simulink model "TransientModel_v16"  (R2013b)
settings: Solver=ode4  StartTime=0.0  StopTime=1500  FixedStep=0.001  RelTol=1e-3
InitFcn:
  | Init_model
StopFcn:
  | Postprocessing2
  | %export_results
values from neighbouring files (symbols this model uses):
  dP = (0:0.005:1)'    [CurveFit_v6_trans.m]
  dP_drag = (0:0.005:1)'    [CurveFit_v6_drag.m]
  Pboost_vec_spd = n_un    [Init_steady_maps.m]
  Pboost_vec_Thr = M_un    [Init_steady_maps.m]
  Pedal = 90    [CurveFit_v6_drag.m]    (also in CurveFit_v6_trans.m = 0:10:90)
  t_sample = 0.01    [Init_model.m]
  time_dy = 0:0.01:5    [CurveFit_v6_drag.m]    (also in CurveFit_v6_trans.m = 0:0.01:10)
undefined symbols (not defined in the file or in its folder): dtaf_sub, dtMbu_sub, dtmf_sub, dtPboost_sub, dtSpeed_Turb_sub, dY, dY_af, dY_af_drag, dY_drag, dY_Mbu, dY_Mbu_drag, dY_mf, dY_mf_drag, dY_Speed_Turb, dY_Speed_Turb_drag, EngineSpeed, EngineSpeed_vec_LM, Mbu_sub_end, Mode, Pboost_Matrix, Speed, Table, Throttle_init, time_dP, time_dP_drag, time_dy_drag, Time_LM, Time_simple, Time_SM, Time_vec_LM
libraries: simulink x45, simulink_extras x4
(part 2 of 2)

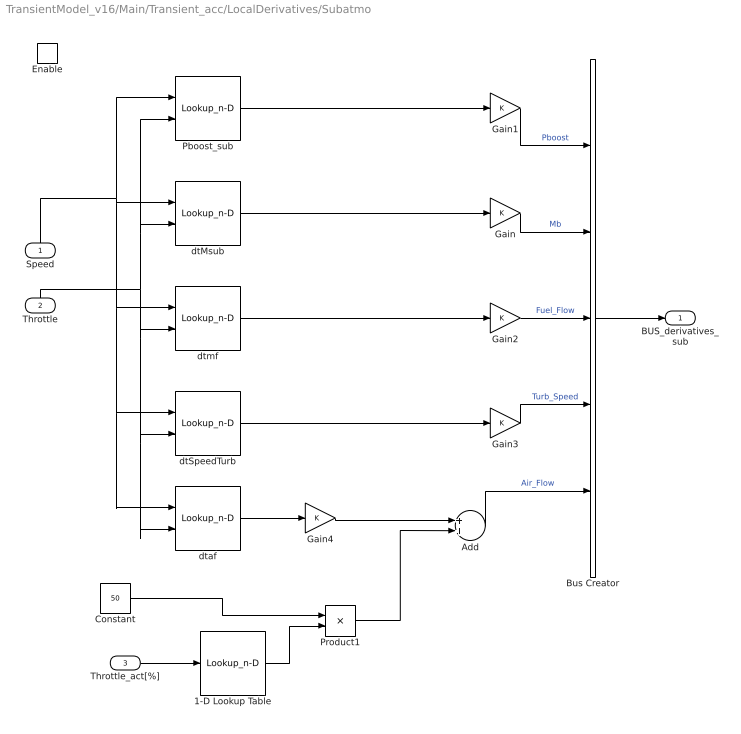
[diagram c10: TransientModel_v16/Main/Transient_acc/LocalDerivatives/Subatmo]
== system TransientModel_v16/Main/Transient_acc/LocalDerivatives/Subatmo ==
  Speed : Inport
  Throttle : Inport  Port=2
  Throttle_act[%] : Inport  Port=3
  Enable : EnablePort  StatesWhenEnabling=reset
  1-D Lookup Table : Lookup_n-D  NumberOfTableDimensions=1  BreakpointsForDimension1=[0,70,75,100]  Table=[50,50,0,0]  InternalRulePriority=Speed  RndMeth=Simplest
  Add : Sum
  Bus Creator : BusCreator  Inputs=5
  Constant : Constant  Value=50
  Gain{,1..4} (5 alike) : Gain
  Pboost_sub : Lookup_n-D  BreakpointsForDimension1=Speed  BreakpointsForDimension2=Pedal  BreakpointsForDimension3=Pedal  Table=dtPboost_sub  ExtrapMethod=Clip  UseLastTableValue=on  RndMeth=Simplest
  Product1 : Product
  dtMsub : Lookup_n-D  BreakpointsForDimension1=Speed  BreakpointsForDimension2=Pedal  BreakpointsForDimension3=Pedal  Table=dtMbu_sub  ExtrapMethod=Clip  UseLastTableValue=on  RndMeth=Simplest
  dtSpeedTurb : Lookup_n-D  BreakpointsForDimension1=Speed  BreakpointsForDimension2=Pedal  BreakpointsForDimension3=Pedal  Table=dtSpeed_Turb_sub  ExtrapMethod=Clip  UseLastTableValue=on  RndMeth=Simplest
  dtaf : Lookup_n-D  BreakpointsForDimension1=Speed  BreakpointsForDimension2=Pedal  BreakpointsForDimension3=Pedal  Table=dtaf_sub  ExtrapMethod=Clip  UseLastTableValue=on  RndMeth=Simplest
  dtmf : Lookup_n-D  BreakpointsForDimension1=Speed  BreakpointsForDimension2=Pedal  BreakpointsForDimension3=Pedal  Table=dtmf_sub  ExtrapMethod=Clip  UseLastTableValue=on  RndMeth=Simplest
  BUS_derivatives_sub : Outport
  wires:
  Throttle/1 -> dtaf/2, dtSpeedTurb/2, dtmf/2, Pboost_sub/2, dtMsub/2
  Speed/1 -> dtaf/1, dtSpeedTurb/1, dtmf/1, dtMsub/1, Pboost_sub/1
  Gain1/1 -> Bus Creator/1  "Pboost"
  Gain/1 -> Bus Creator/2  "Mb"
  Gain2/1 -> Bus Creator/3  "Fuel_Flow"
  Gain3/1 -> Bus Creator/4  "Turb_Speed"
  Pboost_sub/1 -> Gain1/1
  dtMsub/1 -> Gain/1
  dtmf/1 -> Gain2/1
  dtSpeedTurb/1 -> Gain3/1
  Bus Creator/1 -> BUS_derivatives_sub/1
  Add/1 -> Bus Creator/5  "Air_Flow"
  dtaf/1 -> Gain4/1
  Gain4/1 -> Add/1
  Throttle_act[%]/1 -> 1-D Lookup Table/1
  1-D Lookup Table/1 -> Product1/2
  Constant/1 -> Product1/1
  Product1/1 -> Add/2

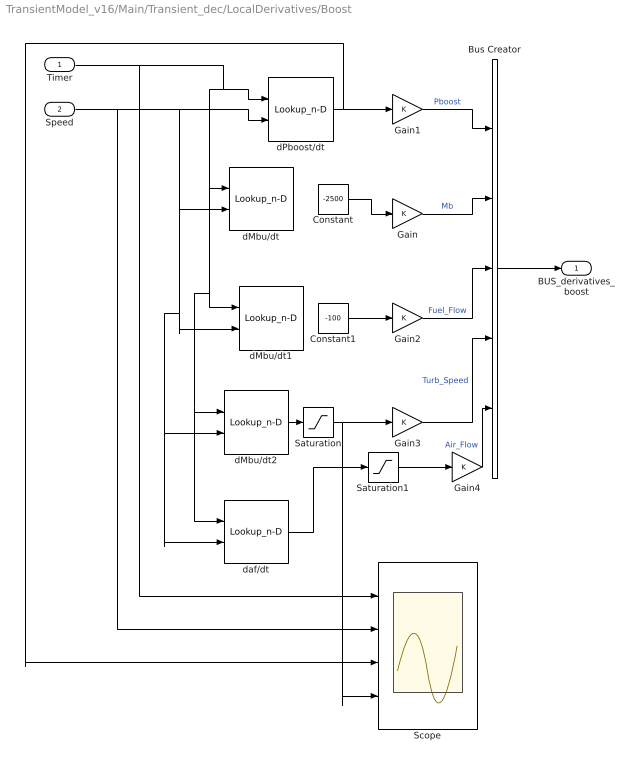
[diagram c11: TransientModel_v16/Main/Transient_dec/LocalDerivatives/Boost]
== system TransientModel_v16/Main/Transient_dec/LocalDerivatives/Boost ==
  Timer : Inport
  Speed : Inport  Port=2
  Bus Creator : BusCreator  Inputs=5
  Constant : Constant  Value=-2500
  Constant1 : Constant  Value=-100
  Gain{,1..4} (5 alike) : Gain
  Saturation : Saturate  UpperLimit=-1000  LowerLimit=-inf
  Saturation1 : Saturate  UpperLimit=-50  LowerLimit=-inf
  Scope : Scope  NumInputPorts=4
  dMbu/dt : Lookup_n-D  BreakpointsForDimension1=time_dy_drag  BreakpointsForDimension2=Speed  BreakpointsForDimension3=Pedal  Table=dY_Mbu_drag  ExtrapMethod=Clip  UseLastTableValue=on  RndMeth=Simplest
  dMbu/dt1 : Lookup_n-D  BreakpointsForDimension1=time_dy_drag  BreakpointsForDimension2=Speed  BreakpointsForDimension3=Pedal  Table=dY_mf_drag  ExtrapMethod=Clip  UseLastTableValue=on  RndMeth=Simplest
  dMbu/dt2 : Lookup_n-D  BreakpointsForDimension1=time_dy_drag  BreakpointsForDimension2=Speed  BreakpointsForDimension3=Pedal  Table=dY_Speed_Turb_drag  ExtrapMethod=Clip  UseLastTableValue=on  RndMeth=Simplest
  dPboost/dt : Lookup_n-D  BreakpointsForDimension1=time_dy_drag  BreakpointsForDimension2=Speed  BreakpointsForDimension3=Pedal  Table=dY_drag  ExtrapMethod=Clip  UseLastTableValue=on  RndMeth=Simplest
  daf/dt : Lookup_n-D  BreakpointsForDimension1=time_dy_drag  BreakpointsForDimension2=Speed  BreakpointsForDimension3=Pedal  Table=dY_af_drag  ExtrapMethod=Clip  UseLastTableValue=on  RndMeth=Simplest
  BUS_derivatives_boost : Outport
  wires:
  dMbu/dt2/1 -> Saturation/1
  dPboost/dt/1 -> Scope/3, Gain1/1
  Bus Creator/1 -> BUS_derivatives_boost/1
  Gain3/1 -> Bus Creator/4  "Turb_Speed"
  Gain2/1 -> Bus Creator/3  "Fuel_Flow"
  Gain/1 -> Bus Creator/2  "Mb"
  Gain1/1 -> Bus Creator/1  "Pboost"
  Timer/1 -> Scope/1, dPboost/dt/1, dMbu/dt/1, dMbu/dt1/1, daf/dt/1, dMbu/dt2/1
  Speed/1 -> Scope/2, dMbu/dt/2, dMbu/dt1/2, daf/dt/2, dMbu/dt2/2, dPboost/dt/2
  Constant/1 -> Gain/1
  Constant1/1 -> Gain2/1
  Saturation/1 -> Scope/4, Gain3/1
  Gain4/1 -> Bus Creator/5  "Air_Flow"
  daf/dt/1 -> Saturation1/1
  Saturation1/1 -> Gain4/1
